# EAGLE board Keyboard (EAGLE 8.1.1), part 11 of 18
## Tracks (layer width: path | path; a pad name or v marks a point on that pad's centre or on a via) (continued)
S$11029 (continued)
  Bottom 0: 44.44,41.74 44.79,41.73
S$11030
  Bottom 0: 44.79,41.73 45.13,41.79
S$11031
  Bottom 0: 45.13,41.79 45.31,41.88
S$11032
  Bottom 0: 45.31,41.88 51,36.2
S$11033
  Bottom 0: 51,36.2 51.05,36.16
S$11034
  Bottom 0: 51.05,36.16 51.11,36.12
S$11035
  Bottom 0: 51.11,36.12 51.17,36.09
S$11036
  Bottom 0: 51.17,36.09 51.24,36.08
S$11037
  Bottom 0: 51.24,36.08 51.31,36.07
S$11038
  Bottom 0: 51.31,36.07 53.88,36.07
S$11039
  Bottom 0: 53.88,36.07 53.83,36.06
S$11040
  Bottom 0: 53.83,36.06 53.54,35.91
S$11041
  Bottom 0: 53.54,35.91 53.31,35.69
S$11042
  Bottom 0: 53.31,35.69 53.13,35.41
S$11043
  Bottom 0: 53.13,35.41 53.05,35.1
S$11044
  Bottom 0: 53.05,35.1 53.05,34.77
S$11045
  Bottom 0: 53.05,34.77 53.13,34.46
S$11046
  Bottom 0: 53.13,34.46 53.31,34.19
S$11047
  Bottom 0: 53.31,34.19 53.54,33.96
S$11048
  Bottom 0: 53.54,33.96 53.83,33.81
S$11049
  Bottom 0: 53.83,33.81 54.15,33.75
S$11050
  Bottom 0: 54.15,33.75 54.48,33.77
S$11051
  Bottom 0: 54.48,33.77 54.57,33.8
S$11052
  Bottom 0: 54.57,33.8 57.92,30.45
S$11053
  Bottom 0: 57.92,30.45 57.92,18.78
S$11054
  Bottom 0: 57.92,18.78 57.92,18.69
S$11055
  Bottom 0: 57.92,18.69 57.95,18.6
S$11056
  Bottom 0: 57.95,18.6 57.98,18.52
S$11057
  Bottom 0: 57.98,18.52 58.03,18.44
S$11058
  Bottom 0: 58.03,18.44 58.09,18.38
S$11059
  Bottom 0: 58.09,18.38 60.24,16.22
S$11060
  Bottom 0: 60.24,16.22 60.2,16.05
S$11061
  Bottom 0: 60.2,16.05 60.2,15.72
S$11062
  Bottom 0: 60.2,15.72 60.28,15.41
S$11063
  Bottom 0: 60.28,15.41 60.45,15.14
S$11064
  Bottom 0: 60.45,15.14 60.69,14.91
S$11065
  Bottom 0: 60.69,14.91 60.81,14.85
S$11066
  Bottom 0: 60.81,14.85 60.81,13.35
S$11067
  Bottom 0: 60.81,13.35 59.95,12.5
S$11068
  Bottom 0: 48.26,30.54 50.03,30.54
S$11069
  Bottom 0: 50.03,30.54 50.11,30.55
S$11070
  Bottom 0: 50.11,30.55 50.18,30.59
S$11071
  Bottom 0: 50.18,30.59 50.24,30.65
S$11072
  Bottom 0: 50.24,30.65 50.28,30.72
S$11073
  Bottom 0: 50.28,30.72 50.29,30.8
S$11074
  Bottom 0: 50.29,30.8 50.29,32.58
S$11075
  Bottom 0: 50.29,32.58 50.28,32.65
S$11076
  Bottom 0: 50.28,32.65 50.24,32.72
S$11077
  Bottom 0: 50.24,32.72 50.18,32.78
S$11078
  Bottom 0: 50.18,32.78 50.11,32.82
S$11079
  Bottom 0: 50.11,32.82 50.03,32.83
S$11080
  Bottom 0: 50.03,32.83 49.59,32.83
S$11081
  Bottom 0: 49.59,32.83 49.59,32.96
S$11082
  Bottom 0: 49.59,32.96 49.53,33.18
S$11083
  Bottom 0: 49.53,33.18 49.37,33.34
S$11084
  Bottom 0: 49.37,33.34 49.15,33.4
S$11085
  Bottom 0: 49.15,33.4 48.78,33.4
S$11086
  Bottom 0: 48.78,33.4 47.7,34.48
S$11087
  Bottom 0: 47.7,34.48 47.76,34.62
S$11088
  Bottom 0: 47.76,34.62 47.8,34.94
S$11089
  Bottom 0: 47.8,34.94 47.76,35.26
S$11090
  Bottom 0: 47.76,35.26 47.63,35.56
S$11091
  Bottom 0: 47.63,35.56 47.42,35.81
S$11092
  Bottom 0: 47.42,35.81 47.16,36
S$11093
  Bottom 0: 47.16,36 46.85,36.11
S$11094
  Bottom 0: 46.85,36.11 46.53,36.13
S$11095
  Bottom 0: 46.53,36.13 46.21,36.06
S$11096
  Bottom 0: 46.21,36.06 45.92,35.91
S$11097
  Bottom 0: 45.92,35.91 45.69,35.69
S$11098
  Bottom 0: 45.69,35.69 45.51,35.41
S$11099
  Bottom 0: 45.51,35.41 45.43,35.1
S$11100
  Bottom 0: 45.43,35.1 45.43,34.77
S$11101
  Bottom 0: 45.43,34.77 45.51,34.46
S$11102
  Bottom 0: 45.51,34.46 45.69,34.19
S$11103
  Bottom 0: 45.69,34.19 45.92,33.96
S$11104
  Bottom 0: 45.92,33.96 46.21,33.81
S$11105
  Bottom 0: 46.21,33.81 46.53,33.75
S$11106
  Bottom 0: 46.53,33.75 46.85,33.77
S$11107
  Bottom 0: 46.85,33.77 47.07,33.85
S$11108
  Bottom 0: 47.07,33.85 48.13,32.79
S$11109
  Bottom 0: 48.13,32.79 48.11,32.78
S$11110
  Bottom 0: 48.11,32.78 48.05,32.72
S$11111
  Bottom 0: 48.05,32.72 48.01,32.65
S$11112
  Bottom 0: 48.01,32.65 48,32.58
S$11113
  Bottom 0: 48,32.58 48,30.8
S$11114
  Bottom 0: 48,30.8 48.01,30.72
S$11115
  Bottom 0: 48.01,30.72 48.05,30.65
S$11116
  Bottom 0: 48.05,30.65 48.11,30.59
S$11117
  Bottom 0: 48.11,30.59 48.18,30.55
S$11118
  Bottom 0: 48.18,30.55 48.26,30.54
S$11119
  Bottom 0: 57.49,39.19 57.84,39.25
S$11120
  Bottom 0: 57.84,39.25 58.15,39.4
S$11121
  Bottom 0: 58.15,39.4 58.42,39.62
S$11122
  Bottom 0: 58.42,39.62 58.63,39.91
S$11123
  Bottom 0: 58.63,39.91 58.76,40.23
S$11124
  Bottom 0: 58.76,40.23 58.8,40.58
S$11125
  Bottom 0: 58.8,40.58 58.76,40.92
S$11126
  Bottom 0: 58.76,40.92 58.63,41.25
S$11127
  Bottom 0: 58.63,41.25 58.42,41.53
S$11128
  Bottom 0: 58.42,41.53 58.15,41.76
S$11129
  Bottom 0: 58.15,41.76 57.84,41.91
S$11130
  Bottom 0: 57.84,41.91 57.49,41.97
S$11131
  Bottom 0: 57.49,41.97 57.14,41.95
S$11132
  Bottom 0: 57.14,41.95 56.81,41.84
S$11133
  Bottom 0: 56.81,41.84 56.78,41.82
S$11134
  Bottom 0: 56.78,41.82 56.2,42.4
S$11135
  Bottom 0: 56.2,42.4 56.16,42.43
S$11136
  Bottom 0: 56.16,42.43 56.1,42.48
S$11137
  Bottom 0: 56.1,42.48 56.03,42.5
S$11138
  Bottom 0: 56.03,42.5 55.97,42.52
S$11139
  Bottom 0: 55.97,42.52 55.9,42.52
S$11140
  Bottom 0: 55.9,42.52 51.33,42.52
S$11141
  Bottom 0: 51.33,42.52 51.26,42.65
S$11142
  Bottom 0: 51.26,42.65 51.06,42.87
S$11143
  Bottom 0: 51.06,42.87 50.79,43.02
S$11144
  Bottom 0: 50.79,43.02 50.49,43.09
S$11145
  Bottom 0: 50.49,43.09 50.19,43.07
S$11146
  Bottom 0: 50.19,43.07 49.91,42.96
S$11147
  Bottom 0: 49.91,42.96 49.67,42.77
S$11148
  Bottom 0: 49.67,42.77 49.51,42.52
S$11149
  Bottom 0: 49.51,42.52 49.41,42.23
S$11150
  Bottom 0: 49.41,42.23 49.41,41.92
S$11151
  Bottom 0: 49.41,41.92 49.51,41.64
S$11152
  Bottom 0: 49.51,41.64 49.67,41.39
S$11153
  Bottom 0: 49.67,41.39 49.91,41.2
S$11154
  Bottom 0: 49.91,41.2 50.19,41.09
S$11155
  Bottom 0: 50.19,41.09 50.49,41.07
S$11156
  Bottom 0: 50.49,41.07 50.79,41.13
S$11157
  Bottom 0: 50.79,41.13 51.06,41.28
S$11158
  Bottom 0: 51.06,41.28 51.26,41.51
S$11159
  Bottom 0: 51.26,41.51 51.33,41.64
S$11160
  Bottom 0: 51.33,41.64 55.72,41.64
S$11161
  Bottom 0: 55.72,41.64 56.16,41.19
S$11162
  Bottom 0: 56.16,41.19 56.11,41.09
S$11163
  Bottom 0: 56.11,41.09 56.02,40.75
S$11164
  Bottom 0: 56.02,40.75 56.02,40.4
S$11165
  Bottom 0: 56.02,40.4 56.11,40.06
S$11166
  Bottom 0: 56.11,40.06 56.28,39.75
S$11167
  Bottom 0: 56.28,39.75 56.52,39.5
S$11168
  Bottom 0: 56.52,39.5 56.81,39.31
S$11169
  Bottom 0: 56.81,39.31 57.14,39.2
S$11170
  Bottom 0: 57.14,39.2 57.49,39.19
S$11171
  Bottom 0: 83.84,60.12 84.13,60.19
S$11172
  Bottom 0: 84.13,60.19 84.4,60.34
S$11173
  Bottom 0: 84.4,60.34 84.6,60.56
S$11174
  Bottom 0: 84.6,60.56 84.73,60.83
S$11175
  Bottom 0: 84.73,60.83 84.78,61.13
S$11176
  Bottom 0: 84.78,61.13 84.73,61.43
S$11177
  Bottom 0: 84.73,61.43 84.6,61.7
S$11178
  Bottom 0: 84.6,61.7 84.4,61.92
S$11179
  Bottom 0: 84.4,61.92 84.13,62.08
S$11180
  Bottom 0: 84.13,62.08 83.84,62.14
S$11181
  Bottom 0: 83.84,62.14 83.53,62.12
S$11182
  Bottom 0: 83.53,62.12 83.25,62.01
S$11183
  Bottom 0: 83.25,62.01 83.02,61.82
S$11184
  Bottom 0: 83.02,61.82 82.84,61.57
S$11185
  Bottom 0: 82.84,61.57 82.75,61.28
S$11186
  Bottom 0: 82.75,61.28 82.75,60.98
S$11187
  Bottom 0: 82.75,60.98 82.84,60.69
S$11188
  Bottom 0: 82.84,60.69 83.02,60.44
S$11189
  Bottom 0: 83.02,60.44 83.25,60.25
S$11190
  Bottom 0: 83.25,60.25 83.53,60.14
S$11191
  Bottom 0: 83.53,60.14 83.84,60.12
S$11192
  Bottom 0: 72.07,68.64 73.85,68.64
S$11193
  Bottom 0: 73.85,68.64 73.92,68.65
S$11194
  Bottom 0: 73.92,68.65 74,68.69
S$11195
  Bottom 0: 74,68.69 74.05,68.75
S$11196
  Bottom 0: 74.05,68.75 74.09,68.82
S$11197
  Bottom 0: 74.09,68.82 74.11,68.9
S$11198
  Bottom 0: 74.11,68.9 74.11,70.67
S$11199
  Bottom 0: 74.11,70.67 74.09,70.75
S$11200
  Bottom 0: 74.09,70.75 74.05,70.82
S$11201
  Bottom 0: 74.05,70.82 74,70.88
S$11202
  Bottom 0: 74,70.88 73.92,70.92
S$11203
  Bottom 0: 73.92,70.92 73.85,70.93
S$11204
  Bottom 0: 73.85,70.93 73.4,70.93
S$11205
  Bottom 0: 73.4,70.93 73.4,71.06
S$11206
  Bottom 0: 73.4,71.06 73.34,71.28
S$11207
  Bottom 0: 73.34,71.28 73.18,71.44
S$11208
  Bottom 0: 73.18,71.44 72.96,71.5
S$11209
  Bottom 0: 72.96,71.5 72.6,71.5
S$11210
  Bottom 0: 72.6,71.5 71.51,72.58
S$11211
  Bottom 0: 71.51,72.58 71.57,72.72
S$11212
  Bottom 0: 71.57,72.72 71.62,73.04
S$11213
  Bottom 0: 71.62,73.04 71.57,73.36
S$11214
  Bottom 0: 71.57,73.36 71.44,73.66
S$11215
  Bottom 0: 71.44,73.66 71.24,73.92
S$11216
  Bottom 0: 71.24,73.92 70.97,74.11
S$11217
  Bottom 0: 70.97,74.11 70.67,74.21
S$11218
  Bottom 0: 70.67,74.21 70.34,74.23
S$11219
  Bottom 0: 70.34,74.23 70.03,74.17
S$11220
  Bottom 0: 70.03,74.17 69.73,74.02
S$11221
  Bottom 0: 69.73,74.02 69.5,73.8
S$11222
  Bottom 0: 69.5,73.8 69.33,73.52
S$11223
  Bottom 0: 69.33,73.52 69.24,73.2
S$11224
  Bottom 0: 69.24,73.2 69.24,72.88
S$11225
  Bottom 0: 69.24,72.88 69.33,72.56
S$11226
  Bottom 0: 69.33,72.56 69.5,72.29
S$11227
  Bottom 0: 69.5,72.29 69.73,72.07
S$11228
  Bottom 0: 69.73,72.07 70.03,71.92
S$11229
  Bottom 0: 70.03,71.92 70.34,71.85
S$11230
  Bottom 0: 70.34,71.85 70.67,71.87
S$11231
  Bottom 0: 70.67,71.87 70.89,71.95
S$11232
  Bottom 0: 70.89,71.95 71.95,70.89
S$11233
  Bottom 0: 71.95,70.89 71.92,70.88
S$11234
  Bottom 0: 71.92,70.88 71.87,70.82
S$11235
  Bottom 0: 71.87,70.82 71.83,70.75
S$11236
  Bottom 0: 71.83,70.75 71.82,70.67
S$11237
  Bottom 0: 71.82,70.67 71.82,68.9
S$11238
  Bottom 0: 71.82,68.9 71.83,68.82
S$11239
  Bottom 0: 71.83,68.82 71.87,68.75
S$11240
  Bottom 0: 71.87,68.75 71.92,68.69
S$11241
  Bottom 0: 71.92,68.69 72,68.65
S$11242
  Bottom 0: 72,68.65 72.07,68.64
S$11243
  Bottom 0: 75.34,68.65 75.66,68.65
S$11244
  Bottom 0: 75.66,68.65 75.97,68.75
S$11245
  Bottom 0: 75.97,68.75 76.25,68.92
S$11246
  Bottom 0: 76.25,68.92 76.46,69.16
S$11247
  Bottom 0: 76.46,69.16 76.6,69.47
S$11248
  Bottom 0: 76.6,69.47 76.64,69.79
S$11249
  Bottom 0: 76.64,69.79 76.6,70.11
S$11250
  Bottom 0: 76.6,70.11 76.46,70.41
S$11251
  Bottom 0: 76.46,70.41 76.25,70.65
S$11252
  Bottom 0: 76.25,70.65 75.97,70.83
S$11253
  Bottom 0: 75.97,70.83 75.66,70.92
S$11254
  Bottom 0: 75.66,70.92 75.34,70.92
S$11255
  Bottom 0: 75.34,70.92 75.03,70.83
S$11256
  Bottom 0: 75.03,70.83 74.75,70.65
S$11257
  Bottom 0: 74.75,70.65 74.54,70.41
S$11258
  Bottom 0: 74.54,70.41 74.4,70.11
S$11259
  Bottom 0: 74.4,70.11 74.36,69.79
S$11260
  Bottom 0: 74.36,69.79 74.4,69.47
S$11261
  Bottom 0: 74.4,69.47 74.54,69.16
S$11262
  Bottom 0: 74.54,69.16 74.75,68.92
S$11263
  Bottom 0: 74.75,68.92 75.03,68.75
S$11264
  Bottom 0: 75.03,68.75 75.34,68.65
S$11265
  Bottom 0: 226.65,12.6 226.66,12.64
S$11266
  Bottom 0: 226.66,12.64 226.62,12.96
S$11267
  Bottom 0: 226.62,12.96 226.48,13.26
S$11268
  Bottom 0: 226.48,13.26 226.27,13.5
S$11269
  Bottom 0: 226.27,13.5 225.99,13.68
S$11270
  Bottom 0: 225.99,13.68 225.68,13.77
S$11271
  Bottom 0: 225.68,13.77 225.57,13.77
S$11272
  Bottom 0: 225.57,13.77 219.4,19.94
S$11273
  Bottom 0: 219.4,19.94 219.34,20
S$11274
  Bottom 0: 219.34,20 219.26,20.04
S$11275
  Bottom 0: 219.26,20.04 219.18,20.08
S$11276
  Bottom 0: 219.18,20.08 219.09,20.1
S$11277
  Bottom 0: 219.09,20.1 219,20.1
S$11278
  Bottom 0: 219,20.1 218.91,20.1
S$11279
  Bottom 0: 218.91,20.1 218.76,20.25
S$11280
  Bottom 0: 218.76,20.25 219.06,20.16
S$11281
  Bottom 0: 219.06,20.16 219.41,20.14
S$11282
  Bottom 0: 219.41,20.14 219.76,20.2
S$11283
  Bottom 0: 219.76,20.2 220.07,20.35
S$11284
  Bottom 0: 220.07,20.35 220.34,20.57
S$11285
  Bottom 0: 220.34,20.57 220.55,20.86
S$11286
  Bottom 0: 220.55,20.86 220.68,21.18
S$11287
  Bottom 0: 220.68,21.18 220.72,21.53
S$11288
  Bottom 0: 220.72,21.53 220.68,21.87
S$11289
  Bottom 0: 220.68,21.87 220.55,22.2
S$11290
  Bottom 0: 220.55,22.2 220.34,22.48
S$11291
  Bottom 0: 220.34,22.48 220.07,22.7
S$11292
  Bottom 0: 220.07,22.7 219.76,22.86
S$11293
  Bottom 0: 219.76,22.86 219.41,22.92
S$11294
  Bottom 0: 219.41,22.92 219.06,22.9
S$11295
  Bottom 0: 219.06,22.9 218.73,22.79
S$11296
  Bottom 0: 218.73,22.79 218.44,22.6
S$11297
  Bottom 0: 218.44,22.6 218.23,22.38
S$11298
  Bottom 0: 218.23,22.38 218.23,25.98
S$11299
  Bottom 0: 218.23,25.98 219.78,27.53
S$11300
  Bottom 0: 219.78,27.53 219.75,27.48
S$11301
  Bottom 0: 219.75,27.48 219.63,27.05
S$11302
  Bottom 0: 219.63,27.05 219.58,26.61
S$11303
  Bottom 0: 219.58,26.61 219.63,26.16
S$11304
  Bottom 0: 219.63,26.16 219.75,25.73
S$11305
  Bottom 0: 219.75,25.73 219.97,25.34
S$11306
  Bottom 0: 219.97,25.34 220.25,24.99
S$11307
  Bottom 0: 220.25,24.99 220.6,24.71
S$11308
  Bottom 0: 220.6,24.71 220.99,24.49
S$11309
  Bottom 0: 220.99,24.49 221.42,24.37
S$11310
  Bottom 0: 221.42,24.37 221.87,24.32
S$11311
  Bottom 0: 221.87,24.32 222.31,24.37
S$11312
  Bottom 0: 222.31,24.37 222.74,24.49
S$11313
  Bottom 0: 222.74,24.49 223.14,24.71
S$11314
  Bottom 0: 223.14,24.71 223.48,24.99
S$11315
  Bottom 0: 223.48,24.99 223.77,25.34
S$11316
  Bottom 0: 223.77,25.34 223.98,25.73
S$11317
  Bottom 0: 223.98,25.73 224.11,26.16
S$11318
  Bottom 0: 224.11,26.16 224.15,26.61
S$11319
  Bottom 0: 224.15,26.61 224.11,27.05
S$11320
  Bottom 0: 224.11,27.05 223.98,27.48
S$11321
  Bottom 0: 223.98,27.48 223.77,27.88
S$11322
  Bottom 0: 223.77,27.88 223.48,28.22
S$11323
  Bottom 0: 223.48,28.22 223.14,28.51
S$11324
  Bottom 0: 223.14,28.51 222.74,28.72
S$11325
  Bottom 0: 222.74,28.72 222.31,28.85
S$11326
  Bottom 0: 222.31,28.85 221.87,28.89
S$11327
  Bottom 0: 221.87,28.89 221.42,28.85
S$11328
  Bottom 0: 221.42,28.85 220.99,28.72
S$11329
  Bottom 0: 220.99,28.72 220.94,28.69
S$11330
  Bottom 0: 220.94,28.69 222.84,30.59
S$11331
  Bottom 0: 222.84,30.59 222.97,30.55
S$11332
  Bottom 0: 222.97,30.55 223.3,30.55
S$11333
  Bottom 0: 223.3,30.55 223.61,30.64
S$11334
  Bottom 0: 223.61,30.64 223.88,30.82
S$11335
  Bottom 0: 223.88,30.82 224.1,31.07
S$11336
  Bottom 0: 224.1,31.07 224.23,31.37
S$11337
  Bottom 0: 224.23,31.37 224.28,31.69
S$11338
  Bottom 0: 224.28,31.69 224.23,32.01
S$11339
  Bottom 0: 224.23,32.01 224.1,32.31
S$11340
  Bottom 0: 224.1,32.31 223.88,32.55
S$11341
  Bottom 0: 223.88,32.55 223.61,32.73
S$11342
  Bottom 0: 223.61,32.73 223.56,32.74
S$11343
  Bottom 0: 223.56,32.74 223.56,33.17
S$11344
  Bottom 0: 223.56,33.17 223.56,33.16
S$11345
  Bottom 0: 223.56,33.16 223.6,33.1
S$11346
  Bottom 0: 223.6,33.1 225.23,31.47
S$11347
  Bottom 0: 225.23,31.47 225.23,25.38
S$11348
  Bottom 0: 225.23,25.38 225.08,25.33
S$11349
  Bottom 0: 225.08,25.33 224.79,25.14
S$11350
  Bottom 0: 224.79,25.14 224.55,24.89
S$11351
  Bottom 0: 224.55,24.89 224.37,24.58
S$11352
  Bottom 0: 224.37,24.58 224.29,24.24
S$11353
  Bottom 0: 224.29,24.24 224.29,23.89
S$11354
  Bottom 0: 224.29,23.89 224.37,23.55
S$11355
  Bottom 0: 224.37,23.55 224.55,23.24
S$11356
  Bottom 0: 224.55,23.24 224.79,22.99
S$11357
  Bottom 0: 224.79,22.99 225.08,22.8
S$11358
  Bottom 0: 225.08,22.8 225.41,22.7
S$11359
  Bottom 0: 225.41,22.7 225.76,22.68
S$11360
  Bottom 0: 225.76,22.68 226.11,22.74
S$11361
  Bottom 0: 226.11,22.74 226.42,22.89
S$11362
  Bottom 0: 226.42,22.89 226.69,23.11
S$11363
  Bottom 0: 226.69,23.11 226.9,23.4
S$11364
  Bottom 0: 226.9,23.4 227.03,23.72
S$11365
  Bottom 0: 227.03,23.72 227.07,24.07
S$11366
  Bottom 0: 227.07,24.07 227.03,24.41
S$11367
  Bottom 0: 227.03,24.41 226.9,24.74
S$11368
  Bottom 0: 226.9,24.74 226.69,25.02
S$11369
  Bottom 0: 226.69,25.02 226.42,25.25
S$11370
  Bottom 0: 226.42,25.25 226.12,25.39
S$11371
  Bottom 0: 226.12,25.39 226.12,31.66
S$11372
  Bottom 0: 226.12,31.66 226.11,31.73
S$11373
  Bottom 0: 226.11,31.73 226.1,31.8
S$11374
  Bottom 0: 226.1,31.8 226.07,31.86
S$11375
  Bottom 0: 226.07,31.86 226.03,31.92
S$11376
  Bottom 0: 226.03,31.92 225.99,31.98
S$11377
  Bottom 0: 225.99,31.98 224.36,33.61
S$11378
  Bottom 0: 224.36,33.61 224.36,36.37
S$11379
  Bottom 0: 224.36,36.37 224.43,36.42
S$11380
  Bottom 0: 224.43,36.42 224.56,36.63
S$11381
  Bottom 0: 224.56,36.63 224.6,36.88
S$11382
  Bottom 0: 224.6,36.88 224.56,37.13
S$11383
  Bottom 0: 224.56,37.13 224.43,37.34
S$11384
  Bottom 0: 224.43,37.34 224.22,37.49
S$11385
  Bottom 0: 224.22,37.49 223.98,37.56
S$11386
  Bottom 0: 223.98,37.56 223.73,37.54
S$11387
  Bottom 0: 223.73,37.54 223.56,37.45
S$11388
  Bottom 0: 223.56,37.45 223.56,38.8
S$11389
  Bottom 0: 223.56,38.8 223.55,38.9
S$11390
  Bottom 0: 223.55,38.9 223.53,38.98
S$11391
  Bottom 0: 223.53,38.98 223.5,39.06
S$11392
  Bottom 0: 223.5,39.06 223.45,39.14
S$11393
  Bottom 0: 223.45,39.14 223.39,39.2
S$11394
  Bottom 0: 223.39,39.2 221.4,41.19
S$11395
  Bottom 0: 221.4,41.19 221.66,41.09
S$11396
  Bottom 0: 221.66,41.09 221.96,41.07
S$11397
  Bottom 0: 221.96,41.07 222.21,41.12
S$11398
  Bottom 0: 222.21,41.12 223.08,40.26
S$11399
  Bottom 0: 223.08,40.26 223.13,40.22
S$11400
  Bottom 0: 223.13,40.22 223.19,40.18
S$11401
  Bottom 0: 223.19,40.18 223.25,40.16
S$11402
  Bottom 0: 223.25,40.16 223.32,40.14
S$11403
  Bottom 0: 223.32,40.14 223.39,40.13
S$11404
  Bottom 0: 223.39,40.13 227.53,40.13
S$11405
  Bottom 0: 227.53,40.13 227.55,40.06
S$11406
  Bottom 0: 227.55,40.06 227.72,39.75
S$11407
  Bottom 0: 227.72,39.75 227.96,39.5
S$11408
  Bottom 0: 227.96,39.5 228.26,39.31
S$11409
  Bottom 0: 228.26,39.31 228.59,39.2
S$11410
  Bottom 0: 228.59,39.2 228.94,39.19
S$11411
  Bottom 0: 228.94,39.19 229.28,39.25
S$11412
  Bottom 0: 229.28,39.25 229.6,39.4
S$11413
  Bottom 0: 229.6,39.4 229.87,39.62
S$11414
  Bottom 0: 229.87,39.62 230.08,39.91
S$11415
  Bottom 0: 230.08,39.91 230.2,40.23
S$11416
  Bottom 0: 230.2,40.23 230.25,40.58
S$11417
  Bottom 0: 230.25,40.58 230.2,40.92
S$11418
  Bottom 0: 230.2,40.92 230.08,41.25
S$11419
  Bottom 0: 230.08,41.25 229.87,41.53
S$11420
  Bottom 0: 229.87,41.53 229.6,41.76
S$11421
  Bottom 0: 229.6,41.76 229.28,41.91
S$11422
  Bottom 0: 229.28,41.91 228.94,41.97
S$11423
  Bottom 0: 228.94,41.97 228.59,41.95
S$11424
  Bottom 0: 228.59,41.95 228.26,41.84
S$11425
  Bottom 0: 228.26,41.84 227.96,41.65
S$11426
  Bottom 0: 227.96,41.65 227.72,41.4
S$11427
  Bottom 0: 227.72,41.4 227.55,41.09
S$11428
  Bottom 0: 227.55,41.09 227.53,41.02
S$11429
  Bottom 0: 227.53,41.02 223.58,41.02
S$11430
  Bottom 0: 223.58,41.02 222.84,41.76
S$11431
  Bottom 0: 222.84,41.76 222.86,41.78
S$11432
  Bottom 0: 222.86,41.78 222.9,42.08
S$11433
  Bottom 0: 222.9,42.08 222.86,42.38
S$11434
  Bottom 0: 222.86,42.38 222.72,42.65
S$11435
  Bottom 0: 222.72,42.65 222.52,42.87
S$11436
  Bottom 0: 222.52,42.87 222.26,43.02
S$11437
  Bottom 0: 222.26,43.02 221.96,43.09
S$11438
  Bottom 0: 221.96,43.09 221.66,43.07
S$11439
  Bottom 0: 221.66,43.07 221.38,42.96
S$11440
  Bottom 0: 221.38,42.96 221.14,42.77
S$11441
  Bottom 0: 221.14,42.77 220.97,42.52
S$11442
  Bottom 0: 220.97,42.52 220.88,42.23
S$11443
  Bottom 0: 220.88,42.23 220.88,41.92
S$11444
  Bottom 0: 220.88,41.92 220.97,41.64
S$11445
  Bottom 0: 220.97,41.64 221,41.59
S$11446
  Bottom 0: 221,41.59 217.79,44.8
S$11447
  Bottom 0: 217.79,44.8 217.79,47.12
S$11448
  Bottom 0: 217.79,47.12 217.79,47.22
S$11449
  Bottom 0: 217.79,47.22 217.76,47.3
S$11450
  Bottom 0: 217.76,47.3 217.73,47.38
S$11451
  Bottom 0: 217.73,47.38 217.69,47.46
S$11452
  Bottom 0: 217.69,47.46 217.62,47.53
S$11453
  Bottom 0: 217.62,47.53 214.71,50.43
S$11454
  Bottom 0: 214.71,50.43 214.75,50.74
S$11455
  Bottom 0: 214.75,50.74 214.71,51.06
S$11456
  Bottom 0: 214.71,51.06 214.57,51.36
S$11457
  Bottom 0: 214.57,51.36 214.36,51.6
S$11458
  Bottom 0: 214.36,51.6 214.08,51.78
S$11459
  Bottom 0: 214.08,51.78 213.77,51.87
S$11460
  Bottom 0: 213.77,51.87 213.45,51.87
S$11461
  Bottom 0: 213.45,51.87 213.14,51.78
S$11462
  Bottom 0: 213.14,51.78 212.87,51.6
S$11463
  Bottom 0: 212.87,51.6 212.65,51.36
S$11464
  Bottom 0: 212.65,51.36 212.51,51.06
S$11465
  Bottom 0: 212.51,51.06 212.47,50.74
S$11466
  Bottom 0: 212.47,50.74 212.51,50.42
S$11467
  Bottom 0: 212.51,50.42 212.65,50.11
S$11468
  Bottom 0: 212.65,50.11 212.87,49.87
S$11469
  Bottom 0: 212.87,49.87 213.14,49.7
S$11470
  Bottom 0: 213.14,49.7 213.45,49.6
S$11471
  Bottom 0: 213.45,49.6 213.77,49.6
S$11472
  Bottom 0: 213.77,49.6 213.9,49.64
S$11473
  Bottom 0: 213.9,49.64 216.65,46.89
S$11474
  Bottom 0: 216.65,46.89 216.65,44.57
S$11475
  Bottom 0: 216.65,44.57 216.66,44.48
S$11476
  Bottom 0: 216.66,44.48 216.68,44.4
S$11477
  Bottom 0: 216.68,44.4 216.59,44.44
S$11478
  Bottom 0: 216.59,44.44 216.59,45.24
S$11479
  Bottom 0: 216.59,45.24 216.59,45.32
S$11480
  Bottom 0: 216.59,45.32 216.57,45.38
S$11481
  Bottom 0: 216.57,45.38 216.55,45.44
S$11482
  Bottom 0: 216.55,45.44 216.51,45.5
S$11483
  Bottom 0: 216.51,45.5 216.47,45.56
S$11484
  Bottom 0: 216.47,45.56 213.65,48.37
S$11485
  Bottom 0: 213.65,48.37 213.6,48.41
S$11486
  Bottom 0: 213.6,48.41 213.53,48.46
S$11487
  Bottom 0: 213.53,48.46 213.47,48.48
S$11488
  Bottom 0: 213.47,48.48 213.41,48.5
S$11489
  Bottom 0: 213.41,48.5 213.34,48.5
S$11490
  Bottom 0: 213.34,48.5 206.52,48.5
S$11491
  Bottom 0: 206.52,48.5 197.68,57.35
S$11492
  Bottom 0: 197.68,57.35 197.62,57.39
S$11493
  Bottom 0: 197.62,57.39 197.56,57.42
S$11494
  Bottom 0: 197.56,57.42 197.5,57.45
S$11495
  Bottom 0: 197.5,57.45 197.43,57.47
S$11496
  Bottom 0: 197.43,57.47 197.36,57.47
S$11497
  Bottom 0: 197.36,57.47 178.6,57.47
S$11498
  Bottom 0: 178.6,57.47 174.54,61.54
S$11499
  Bottom 0: 174.54,61.54 174.64,61.82
S$11500
  Bottom 0: 174.64,61.82 174.69,62.17
S$11501
  Bottom 0: 174.69,62.17 174.64,62.51
S$11502
  Bottom 0: 174.64,62.51 174.52,62.84
S$11503
  Bottom 0: 174.52,62.84 174.31,63.12
S$11504
  Bottom 0: 174.31,63.12 174.13,63.27
S$11505
  Bottom 0: 174.13,63.27 175.71,63.27
S$11506
  Bottom 0: 175.71,63.27 176.99,61.99
S$11507
  Bottom 0: 176.99,61.99 177.04,61.95
S$11508
  Bottom 0: 177.04,61.95 177.1,61.91
S$11509
  Bottom 0: 177.1,61.91 177.16,61.89
S$11510
  Bottom 0: 177.16,61.89 177.23,61.87
S$11511
  Bottom 0: 177.23,61.87 177.3,61.86
S$11512
  Bottom 0: 177.3,61.86 178.33,61.86
S$11513
  Bottom 0: 178.33,61.86 178.27,61.82
S$11514
  Bottom 0: 178.27,61.82 178.11,61.57
S$11515
  Bottom 0: 178.11,61.57 178.01,61.28
S$11516
  Bottom 0: 178.01,61.28 178.01,60.98
S$11517
  Bottom 0: 178.01,60.98 178.11,60.69
S$11518
  Bottom 0: 178.11,60.69 178.27,60.44
S$11519
  Bottom 0: 178.27,60.44 178.51,60.25
S$11520
  Bottom 0: 178.51,60.25 178.79,60.14
S$11521
  Bottom 0: 178.79,60.14 179.09,60.12
S$11522
  Bottom 0: 179.09,60.12 179.39,60.19
S$11523
  Bottom 0: 179.39,60.19 179.66,60.34
S$11524
  Bottom 0: 179.66,60.34 179.86,60.56
S$11525
  Bottom 0: 179.86,60.56 179.92,60.69
S$11526
  Bottom 0: 179.92,60.69 184.3,60.69
S$11527
  Bottom 0: 184.3,60.69 184.74,60.24
S$11528
  Bottom 0: 184.74,60.24 184.69,60.14
S$11529
  Bottom 0: 184.69,60.14 184.6,59.8
S$11530
  Bottom 0: 184.6,59.8 184.6,59.45
S$11531
  Bottom 0: 184.6,59.45 184.69,59.11
S$11532
  Bottom 0: 184.69,59.11 184.86,58.8
S$11533
  Bottom 0: 184.86,58.8 185.1,58.55
S$11534
  Bottom 0: 185.1,58.55 185.4,58.36
S$11535
  Bottom 0: 185.4,58.36 185.73,58.26
S$11536
  Bottom 0: 185.73,58.26 186.07,58.23
S$11537
  Bottom 0: 186.07,58.23 186.42,58.3
S$11538
  Bottom 0: 186.42,58.3 186.74,58.45
S$11539
  Bottom 0: 186.74,58.45 187.01,58.67
S$11540
  Bottom 0: 187.01,58.67 187.22,58.96
S$11541
  Bottom 0: 187.22,58.96 187.34,59.28
S$11542
  Bottom 0: 187.34,59.28 187.39,59.63
S$11543
  Bottom 0: 187.39,59.63 187.34,59.97
S$11544
  Bottom 0: 187.34,59.97 187.22,60.3
S$11545
  Bottom 0: 187.22,60.3 187.01,60.58
S$11546
  Bottom 0: 187.01,60.58 186.74,60.8
S$11547
  Bottom 0: 186.74,60.8 186.42,60.96
S$11548
  Bottom 0: 186.42,60.96 186.07,61.02
S$11549
  Bottom 0: 186.07,61.02 185.73,61
S$11550
  Bottom 0: 185.73,61 185.4,60.89
S$11551
  Bottom 0: 185.4,60.89 185.37,60.87
S$11552
  Bottom 0: 185.37,60.87 184.8,61.45
S$11553
  Bottom 0: 184.8,61.45 184.74,61.48
S$11554
  Bottom 0: 184.74,61.48 184.68,61.53
S$11555
  Bottom 0: 184.68,61.53 184.62,61.55
S$11556
  Bottom 0: 184.62,61.55 184.56,61.57
S$11557
  Bottom 0: 184.56,61.57 184.49,61.57
S$11558
  Bottom 0: 184.49,61.57 179.92,61.57
S$11559
  Bottom 0: 179.92,61.57 179.86,61.7
S$11560
  Bottom 0: 179.86,61.7 179.71,61.86
S$11561
  Bottom 0: 179.71,61.86 190.99,61.86
S$11562
  Bottom 0: 190.99,61.86 191.04,61.65
S$11563
  Bottom 0: 191.04,61.65 191.21,61.34
S$11564
  Bottom 0: 191.21,61.34 191.45,61.09
S$11565
  Bottom 0: 191.45,61.09 191.75,60.9
S$11566
  Bottom 0: 191.75,60.9 192.08,60.8
S$11567
  Bottom 0: 192.08,60.8 192.43,60.77
S$11568
  Bottom 0: 192.43,60.77 192.77,60.84
S$11569
  Bottom 0: 192.77,60.84 193.09,60.99
S$11570
  Bottom 0: 193.09,60.99 193.36,61.21
S$11571
  Bottom 0: 193.36,61.21 193.57,61.5
S$11572
  Bottom 0: 193.57,61.5 193.69,61.82
S$11573
  Bottom 0: 193.69,61.82 193.74,62.17
S$11574
  Bottom 0: 193.74,62.17 193.69,62.51
S$11575
  Bottom 0: 193.69,62.51 193.57,62.84
S$11576
  Bottom 0: 193.57,62.84 193.36,63.12
S$11577
  Bottom 0: 193.36,63.12 193.09,63.34
S$11578
  Bottom 0: 193.09,63.34 192.78,63.49
S$11579
  Bottom 0: 192.78,63.49 192.78,64.65
S$11580
  Bottom 0: 192.78,64.65 197.08,68.95
S$11581
  Bottom 0: 197.08,68.95 197.06,68.9
S$11582
  Bottom 0: 197.06,68.9 197.06,68.59
S$11583
  Bottom 0: 197.06,68.59 197.16,68.31
S$11584
  Bottom 0: 197.16,68.31 197.32,68.06
S$11585
  Bottom 0: 197.32,68.06 197.56,67.87
S$11586
  Bottom 0: 197.56,67.87 197.84,67.76
S$11587
  Bottom 0: 197.84,67.76 198.15,67.74
S$11588
  Bottom 0: 198.15,67.74 198.39,67.8
S$11589
  Bottom 0: 198.39,67.8 205.18,61.01
S$11590
  Bottom 0: 205.18,61.01 205.12,61.02
S$11591
  Bottom 0: 205.12,61.02 204.78,61
S$11592
  Bottom 0: 204.78,61 204.45,60.89
S$11593
  Bottom 0: 204.45,60.89 204.42,60.87
S$11594
  Bottom 0: 204.42,60.87 203.84,61.45
S$11595
  Bottom 0: 203.84,61.45 203.79,61.48
S$11596
  Bottom 0: 203.79,61.48 203.73,61.53
S$11597
  Bottom 0: 203.73,61.53 203.67,61.55
S$11598
  Bottom 0: 203.67,61.55 203.6,61.57
S$11599
  Bottom 0: 203.6,61.57 203.53,61.57
S$11600
  Bottom 0: 203.53,61.57 198.97,61.57
S$11601
  Bottom 0: 198.97,61.57 198.91,61.7
S$11602
  Bottom 0: 198.91,61.7 198.71,61.92
S$11603
  Bottom 0: 198.71,61.92 198.44,62.08
S$11604
  Bottom 0: 198.44,62.08 198.15,62.14
S$11605
  Bottom 0: 198.15,62.14 197.84,62.12
S$11606
  Bottom 0: 197.84,62.12 197.56,62.01
S$11607
  Bottom 0: 197.56,62.01 197.32,61.82
S$11608
  Bottom 0: 197.32,61.82 197.16,61.57
S$11609
  Bottom 0: 197.16,61.57 197.06,61.28
S$11610
  Bottom 0: 197.06,61.28 197.06,60.98
S$11611
  Bottom 0: 197.06,60.98 197.16,60.69
S$11612
  Bottom 0: 197.16,60.69 197.32,60.44
S$11613
  Bottom 0: 197.32,60.44 197.56,60.25
S$11614
  Bottom 0: 197.56,60.25 197.84,60.14
S$11615
  Bottom 0: 197.84,60.14 198.15,60.12
S$11616
  Bottom 0: 198.15,60.12 198.44,60.19
S$11617
  Bottom 0: 198.44,60.19 198.71,60.34
S$11618
  Bottom 0: 198.71,60.34 198.91,60.56
S$11619
  Bottom 0: 198.91,60.56 198.97,60.69
S$11620
  Bottom 0: 198.97,60.69 203.35,60.69
S$11621
  Bottom 0: 203.35,60.69 203.79,60.24
S$11622
  Bottom 0: 203.79,60.24 203.74,60.14
S$11623
  Bottom 0: 203.74,60.14 203.66,59.8
S$11624
  Bottom 0: 203.66,59.8 203.66,59.45
S$11625
  Bottom 0: 203.66,59.45 203.74,59.11
S$11626
  Bottom 0: 203.74,59.11 203.91,58.8
S$11627
  Bottom 0: 203.91,58.8 204.15,58.55
S$11628
  Bottom 0: 204.15,58.55 204.45,58.36
S$11629
  Bottom 0: 204.45,58.36 204.78,58.26
S$11630
  Bottom 0: 204.78,58.26 205.12,58.23
S$11631
  Bottom 0: 205.12,58.23 205.47,58.3
S$11632
  Bottom 0: 205.47,58.3 205.79,58.45
S$11633
  Bottom 0: 205.79,58.45 206.06,58.67
S$11634
  Bottom 0: 206.06,58.67 206.27,58.96
S$11635
  Bottom 0: 206.27,58.96 206.39,59.28
S$11636
  Bottom 0: 206.39,59.28 206.44,59.63
S$11637
  Bottom 0: 206.44,59.63 206.42,59.77
S$11638
  Bottom 0: 206.42,59.77 223.95,42.24
S$11639
  Bottom 0: 223.95,42.24 224,42.2
S$11640
  Bottom 0: 224,42.2 224.07,42.16
S$11641
  Bottom 0: 224.07,42.16 224.13,42.14
S$11642
  Bottom 0: 224.13,42.14 224.19,42.12
S$11643
  Bottom 0: 224.19,42.12 224.26,42.11
S$11644
  Bottom 0: 224.26,42.11 232.72,42.11
S$11645
  Bottom 0: 232.72,42.11 233.54,41.29
S$11646
  Bottom 0: 233.54,41.29 233.6,41.25
S$11647
  Bottom 0: 233.6,41.25 233.66,41.21
S$11648
  Bottom 0: 233.66,41.21 233.72,41.19
S$11649
  Bottom 0: 233.72,41.19 233.78,41.17
S$11650
  Bottom 0: 233.78,41.17 233.85,41.16
S$11651
  Bottom 0: 233.85,41.16 235.85,41.16
S$11652
  Bottom 0: 235.85,41.16 235.92,41.17
S$11653
  Bottom 0: 235.92,41.17 235.98,41.19
S$11654
  Bottom 0: 235.98,41.19 236.04,41.21
S$11655
  Bottom 0: 236.04,41.21 236.11,41.25
S$11656
  Bottom 0: 236.11,41.25 236.16,41.29
S$11657
  Bottom 0: 236.16,41.29 242.93,48.06
S$11658
  Bottom 0: 242.93,48.06 242.97,48.12
S$11659
  Bottom 0: 242.97,48.12 243.01,48.17
S$11660
  Bottom 0: 243.01,48.17 243.04,48.24
S$11661
  Bottom 0: 243.04,48.24 243.06,48.3
S$11662
  Bottom 0: 243.06,48.3 243.06,48.35
S$11663
  Bottom 0: 243.06,48.35 243.13,48.4
S$11664
  Bottom 0: 243.13,48.4 243.26,48.62
S$11665
  Bottom 0: 243.26,48.62 243.3,48.87
S$11666
  Bottom 0: 243.3,48.87 243.26,49.12
S$11667
  Bottom 0: 243.26,49.12 243.25,49.13
S$11668
  Bottom 0: 243.25,49.13 243.47,49.18
S$11669
  Bottom 0: 243.47,49.18 243.52,49.22
S$11670
  Bottom 0: 243.52,49.22 243.52,29.46
S$11671
  Bottom 0: 243.52,29.46 226.65,12.6
S$11672
  Bottom 0: 228,14.7 228.33,14.72
S$11673
  Bottom 0: 228.33,14.72 228.63,14.83
S$11674
  Bottom 0: 228.63,14.83 228.9,15.01
S$11675
  Bottom 0: 228.9,15.01 229.1,15.27
S$11676
  Bottom 0: 229.1,15.27 229.23,15.57
S$11677
  Bottom 0: 229.23,15.57 229.28,15.89
S$11678
  Bottom 0: 229.28,15.89 229.23,16.21
S$11679
  Bottom 0: 229.23,16.21 229.1,16.51
S$11680
  Bottom 0: 229.1,16.51 228.9,16.76
S$11681
  Bottom 0: 228.9,16.76 228.65,16.93
S$11682
  Bottom 0: 228.65,16.93 228.65,28.03
S$11683
  Bottom 0: 228.65,28.03 229.89,29.27
S$11684
  Bottom 0: 229.89,29.27 230.14,29.22
S$11685
  Bottom 0: 230.14,29.22 230.46,29.24
S$11686
  Bottom 0: 230.46,29.24 230.77,29.35
S$11687
  Bottom 0: 230.77,29.35 231.03,29.54
S$11688
  Bottom 0: 231.03,29.54 231.24,29.79
S$11689
  Bottom 0: 231.24,29.79 231.37,30.09
S$11690
  Bottom 0: 231.37,30.09 231.41,30.41
S$11691
  Bottom 0: 231.41,30.41 231.37,30.73
S$11692
  Bottom 0: 231.37,30.73 231.24,31.03
S$11693
  Bottom 0: 231.24,31.03 231.03,31.29
S$11694
  Bottom 0: 231.03,31.29 230.77,31.47
S$11695
  Bottom 0: 230.77,31.47 230.46,31.58
S$11696
  Bottom 0: 230.46,31.58 230.14,31.6
S$11697
  Bottom 0: 230.14,31.6 229.89,31.55
S$11698
  Bottom 0: 229.89,31.55 226.84,34.6
S$11699
  Bottom 0: 226.84,34.6 226.85,34.62
S$11700
  Bottom 0: 226.85,34.62 226.9,34.94
S$11701
  Bottom 0: 226.9,34.94 226.85,35.26
S$11702
  Bottom 0: 226.85,35.26 226.72,35.56
S$11703
  Bottom 0: 226.72,35.56 226.51,35.81
S$11704
  Bottom 0: 226.51,35.81 226.25,36
S$11705
  Bottom 0: 226.25,36 225.95,36.11
S$11706
  Bottom 0: 225.95,36.11 225.62,36.13
S$11707
  Bottom 0: 225.62,36.13 225.3,36.06
S$11708
  Bottom 0: 225.3,36.06 225.01,35.91
S$11709
  Bottom 0: 225.01,35.91 224.78,35.69
S$11710
  Bottom 0: 224.78,35.69 224.6,35.41
S$11711
  Bottom 0: 224.6,35.41 224.52,35.1
S$11712
  Bottom 0: 224.52,35.1 224.52,34.77
S$11713
  Bottom 0: 224.52,34.77 224.6,34.46
S$11714
  Bottom 0: 224.6,34.46 224.78,34.19
S$11715
  Bottom 0: 224.78,34.19 225.01,33.96
S$11716
  Bottom 0: 225.01,33.96 225.3,33.81
S$11717
  Bottom 0: 225.3,33.81 225.62,33.75
S$11718
  Bottom 0: 225.62,33.75 225.95,33.77
S$11719
  Bottom 0: 225.95,33.77 226.04,33.8
S$11720
  Bottom 0: 226.04,33.8 229.09,30.75
S$11721
  Bottom 0: 229.09,30.75 229.04,30.57
S$11722
  Bottom 0: 229.04,30.57 229.04,30.25
S$11723
  Bottom 0: 229.04,30.25 229.09,30.08
S$11724
  Bottom 0: 229.09,30.08 227.68,28.67
S$11725
  Bottom 0: 227.68,28.67 227.62,28.6
S$11726
  Bottom 0: 227.62,28.6 227.58,28.53
S$11727
  Bottom 0: 227.58,28.53 227.54,28.45
S$11728
  Bottom 0: 227.54,28.45 227.52,28.35
S$11729
  Bottom 0: 227.52,28.35 227.51,28.27
S$11730
  Bottom 0: 227.51,28.27 227.51,16.92
S$11731
  Bottom 0: 227.51,16.92 227.39,16.86
S$11732
  Bottom 0: 227.39,16.86 227.16,16.64
S$11733
  Bottom 0: 227.16,16.64 226.99,16.36
S$11734
  Bottom 0: 226.99,16.36 226.9,16.05
S$11735
  Bottom 0: 226.9,16.05 226.9,15.72
S$11736
  Bottom 0: 226.9,15.72 226.99,15.41
S$11737
  Bottom 0: 226.99,15.41 227.16,15.14
S$11738
  Bottom 0: 227.16,15.14 227.39,14.91
S$11739
  Bottom 0: 227.39,14.91 227.68,14.77
S$11740
  Bottom 0: 227.68,14.77 228,14.7
S$11741
  Bottom 0: 230.14,21.6 230.46,21.62
S$11742
  Bottom 0: 230.46,21.62 230.77,21.73
S$11743
  Bottom 0: 230.77,21.73 231.03,21.92
S$11744
  Bottom 0: 231.03,21.92 231.24,22.17
S$11745
  Bottom 0: 231.24,22.17 231.32,22.35
S$11746
  Bottom 0: 231.32,22.35 233.03,22.35
S$11747
  Bottom 0: 233.03,22.35 233.1,22.36
S$11748
  Bottom 0: 233.1,22.36 233.17,22.37
S$11749
  Bottom 0: 233.17,22.37 233.23,22.39
S$11750
  Bottom 0: 233.23,22.39 233.29,22.44
S$11751
  Bottom 0: 233.29,22.44 233.35,22.48
S$11752
  Bottom 0: 233.35,22.48 241.89,31.02
S$11753
  Bottom 0: 241.89,31.02 241.99,31.01
S$11754
  Bottom 0: 241.99,31.01 242.23,31.07
S$11755
  Bottom 0: 242.23,31.07 242.44,31.22
S$11756
  Bottom 0: 242.44,31.22 242.57,31.44
S$11757
  Bottom 0: 242.57,31.44 242.61,31.69
S$11758
  Bottom 0: 242.61,31.69 242.57,31.93
S$11759
  Bottom 0: 242.57,31.93 242.44,32.15
S$11760
  Bottom 0: 242.44,32.15 242.23,32.3
S$11761
  Bottom 0: 242.23,32.3 241.99,32.37
S$11762
  Bottom 0: 241.99,32.37 241.74,32.35
S$11763
  Bottom 0: 241.74,32.35 241.51,32.23
S$11764
  Bottom 0: 241.51,32.23 241.34,32.05
S$11765
  Bottom 0: 241.34,32.05 241.25,31.81
S$11766
  Bottom 0: 241.25,31.81 241.25,31.64
S$11767
  Bottom 0: 241.25,31.64 232.84,23.23
S$11768
  Bottom 0: 232.84,23.23 231.32,23.23
S$11769
  Bottom 0: 231.32,23.23 231.24,23.41
S$11770
  Bottom 0: 231.24,23.41 231.03,23.66
S$11771
  Bottom 0: 231.03,23.66 230.77,23.85
S$11772
  Bottom 0: 230.77,23.85 230.46,23.96
S$11773
  Bottom 0: 230.46,23.96 230.14,23.98
S$11774
  Bottom 0: 230.14,23.98 229.82,23.91
S$11775
  Bottom 0: 229.82,23.91 229.53,23.77
S$11776
  Bottom 0: 229.53,23.77 229.3,23.54
S$11777
  Bottom 0: 229.3,23.54 229.13,23.27
S$11778
  Bottom 0: 229.13,23.27 229.04,22.95
S$11779
  Bottom 0: 229.04,22.95 229.04,22.63
S$11780
  Bottom 0: 229.04,22.63 229.13,22.31
S$11781
  Bottom 0: 229.13,22.31 229.3,22.04
S$11782
  Bottom 0: 229.3,22.04 229.53,21.82
S$11783
  Bottom 0: 229.53,21.82 229.82,21.67
S$11784
  Bottom 0: 229.82,21.67 230.14,21.6
S$11785
  Bottom 0: 241.02,41.07 241.31,41.13
S$11786
  Bottom 0: 241.31,41.13 241.57,41.28
S$11787
  Bottom 0: 241.57,41.28 241.78,41.51
S$11788
  Bottom 0: 241.78,41.51 241.91,41.78
S$11789
  Bottom 0: 241.91,41.78 241.96,42.08
S$11790
  Bottom 0: 241.96,42.08 241.91,42.38
S$11791
  Bottom 0: 241.91,42.38 241.78,42.65
S$11792
  Bottom 0: 241.78,42.65 241.57,42.87
S$11793
  Bottom 0: 241.57,42.87 241.31,43.02
S$11794
  Bottom 0: 241.31,43.02 241.02,43.09
S$11795
  Bottom 0: 241.02,43.09 240.71,43.07
S$11796
  Bottom 0: 240.71,43.07 240.43,42.96
S$11797
  Bottom 0: 240.43,42.96 240.19,42.77
S$11798
  Bottom 0: 240.19,42.77 240.03,42.52
S$11799
  Bottom 0: 240.03,42.52 239.94,42.23
S$11800
  Bottom 0: 239.94,42.23 239.94,41.92
S$11801
  Bottom 0: 239.94,41.92 240.03,41.64
S$11802
  Bottom 0: 240.03,41.64 240.19,41.39
S$11803
  Bottom 0: 240.19,41.39 240.43,41.2
S$11804
  Bottom 0: 240.43,41.2 240.71,41.09
S$11805
  Bottom 0: 240.71,41.09 241.02,41.07
S$11806
  Bottom 0: 210.18,49.59 211.96,49.59
S$11807
  Bottom 0: 211.96,49.59 212.04,49.6
S$11808
  Bottom 0: 212.04,49.6 212.11,49.64
S$11809
  Bottom 0: 212.11,49.64 212.16,49.7
S$11810
  Bottom 0: 212.16,49.7 212.2,49.77
S$11811
  Bottom 0: 212.2,49.77 212.21,49.85
S$11812
  Bottom 0: 212.21,49.85 212.21,51.63
S$11813
  Bottom 0: 212.21,51.63 212.2,51.7
S$11814
  Bottom 0: 212.2,51.7 212.16,51.77
S$11815
  Bottom 0: 212.16,51.77 212.11,51.83
S$11816
  Bottom 0: 212.11,51.83 212.04,51.87
S$11817
  Bottom 0: 212.04,51.87 211.96,51.88
S$11818
  Bottom 0: 211.96,51.88 211.51,51.88
S$11819
  Bottom 0: 211.51,51.88 211.51,52.01
S$11820
  Bottom 0: 211.51,52.01 211.45,52.23
S$11821
  Bottom 0: 211.45,52.23 211.29,52.39
S$11822
  Bottom 0: 211.29,52.39 211.07,52.45
S$11823
  Bottom 0: 211.07,52.45 210.72,52.45
S$11824
  Bottom 0: 210.72,52.45 209.64,53.52
S$11825
  Bottom 0: 209.64,53.52 209.7,53.67
S$11826
  Bottom 0: 209.7,53.67 209.75,53.98
S$11827
  Bottom 0: 209.75,53.98 209.7,54.3
S$11828
  Bottom 0: 209.7,54.3 209.57,54.61
S$11829
  Bottom 0: 209.57,54.61 209.37,54.86
S$11830
  Bottom 0: 209.37,54.86 209.1,55.05
S$11831
  Bottom 0: 209.1,55.05 208.8,55.16
S$11832
  Bottom 0: 208.8,55.16 208.47,55.18
S$11833
  Bottom 0: 208.47,55.18 208.15,55.11
S$11834
  Bottom 0: 208.15,55.11 207.86,54.96
S$11835
  Bottom 0: 207.86,54.96 207.63,54.74
S$11836
  Bottom 0: 207.63,54.74 207.45,54.47
S$11837
  Bottom 0: 207.45,54.47 207.37,54.15
S$11838
  Bottom 0: 207.37,54.15 207.37,53.83
S$11839
  Bottom 0: 207.37,53.83 207.45,53.51
S$11840
  Bottom 0: 207.45,53.51 207.63,53.23
S$11841
  Bottom 0: 207.63,53.23 207.86,53.01
S$11842
  Bottom 0: 207.86,53.01 208.15,52.87
S$11843
  Bottom 0: 208.15,52.87 208.47,52.8
S$11844
  Bottom 0: 208.47,52.8 208.8,52.82
S$11845
  Bottom 0: 208.8,52.82 209.02,52.9
S$11846
  Bottom 0: 209.02,52.9 210.07,51.85
S$11847
  Bottom 0: 210.07,51.85 210.03,51.83
S$11848
  Bottom 0: 210.03,51.83 209.98,51.77
S$11849
  Bottom 0: 209.98,51.77 209.94,51.7
S$11850
  Bottom 0: 209.94,51.7 209.93,51.63
S$11851
  Bottom 0: 209.93,51.63 209.93,49.85
S$11852
  Bottom 0: 209.93,49.85 209.94,49.77
S$11853
  Bottom 0: 209.94,49.77 209.98,49.7
S$11854
  Bottom 0: 209.98,49.7 210.03,49.64
S$11855
  Bottom 0: 210.03,49.64 210.11,49.6
S$11856
  Bottom 0: 210.11,49.6 210.18,49.59
S$11857
  Bottom 0: 12.19,13.21 12.17,13.26
S$11858
  Bottom 0: 12.17,13.26 11.95,13.5
S$11859
  Bottom 0: 11.95,13.5 11.68,13.68
S$11860
  Bottom 0: 11.68,13.68 11.37,13.77
S$11861
  Bottom 0: 11.37,13.77 11.05,13.77
S$11862
  Bottom 0: 11.05,13.77 10.73,13.68
S$11863
  Bottom 0: 10.73,13.68 10.46,13.5
S$11864
  Bottom 0: 10.46,13.5 10.37,13.39
S$11865
  Bottom 0: 10.37,13.39 10.37,34.35
S$11866
  Bottom 0: 10.37,34.35 17.89,41.86
S$11867
  Bottom 0: 17.89,41.86 17.91,41.85
S$11868
  Bottom 0: 17.91,41.85 18.24,41.74
S$11869
  Bottom 0: 18.24,41.74 18.59,41.73
S$11870
  Bottom 0: 18.59,41.73 18.94,41.79
S$11871
  Bottom 0: 18.94,41.79 19.26,41.94
S$11872
  Bottom 0: 19.26,41.94 19.52,42.16
S$11873
  Bottom 0: 19.52,42.16 19.68,42.38
S$11874
  Bottom 0: 19.68,42.38 19.68,40.49
S$11875
  Bottom 0: 19.68,40.49 17.65,38.45
S$11876
  Bottom 0: 17.65,38.45 17.56,38.48
S$11877
  Bottom 0: 17.56,38.48 17.24,38.5
S$11878
  Bottom 0: 17.24,38.5 16.92,38.44
S$11879
  Bottom 0: 16.92,38.44 16.63,38.29
S$11880
  Bottom 0: 16.63,38.29 16.4,38.07
S$11881
  Bottom 0: 16.4,38.07 16.22,37.79
S$11882
  Bottom 0: 16.22,37.79 16.13,37.48
S$11883
  Bottom 0: 16.13,37.48 16.13,37.15
S$11884
  Bottom 0: 16.13,37.15 16.22,36.84
S$11885
  Bottom 0: 16.22,36.84 16.4,36.56
S$11886
  Bottom 0: 16.4,36.56 16.63,36.34
S$11887
  Bottom 0: 16.63,36.34 16.92,36.19
S$11888
  Bottom 0: 16.92,36.19 17.24,36.13
S$11889
  Bottom 0: 17.24,36.13 17.56,36.15
S$11890
  Bottom 0: 17.56,36.15 17.87,36.25
S$11891
  Bottom 0: 17.87,36.25 18.13,36.44
S$11892
  Bottom 0: 18.13,36.44 18.34,36.7
S$11893
  Bottom 0: 18.34,36.7 18.47,36.99
S$11894
  Bottom 0: 18.47,36.99 18.51,37.31
S$11895
  Bottom 0: 18.51,37.31 18.47,37.63
S$11896
  Bottom 0: 18.47,37.63 18.46,37.66
S$11897
  Bottom 0: 18.46,37.66 20.66,39.85
S$11898
  Bottom 0: 20.66,39.85 20.72,39.92
S$11899
  Bottom 0: 20.72,39.92 20.77,40
S$11900
  Bottom 0: 20.77,40 20.8,40.08
S$11901
  Bottom 0: 20.8,40.08 20.82,40.16
S$11902
  Bottom 0: 20.82,40.16 20.82,40.26
S$11903
  Bottom 0: 20.82,40.26 20.82,45.55
S$11904
  Bottom 0: 20.82,45.55 20.82,45.65
S$11905
  Bottom 0: 20.82,45.65 20.8,45.73
S$11906
  Bottom 0: 20.8,45.73 20.77,45.81
S$11907
  Bottom 0: 20.77,45.81 20.72,45.89
S$11908
  Bottom 0: 20.72,45.89 20.66,45.96
S$11909
  Bottom 0: 20.66,45.96 17.38,49.24
S$11910
  Bottom 0: 17.38,49.24 17.9,49.77
S$11911
  Bottom 0: 17.9,49.77 17.96,49.83
S$11912
  Bottom 0: 17.96,49.83 18.01,49.91
S$11913
  Bottom 0: 18.01,49.91 18.04,49.99
S$11914
  Bottom 0: 18.04,49.99 18.07,50.08
S$11915
  Bottom 0: 18.07,50.08 18.07,50.17
S$11916
  Bottom 0: 18.07,50.17 18.07,53.07
S$11917
  Bottom 0: 18.07,53.07 18.13,53.11
S$11918
  Bottom 0: 18.13,53.11 18.34,53.37
S$11919
  Bottom 0: 18.34,53.37 18.47,53.67
S$11920
  Bottom 0: 18.47,53.67 18.51,53.98
S$11921
  Bottom 0: 18.51,53.98 18.47,54.3
S$11922
  Bottom 0: 18.47,54.3 18.34,54.61
S$11923
  Bottom 0: 18.34,54.61 18.13,54.86
S$11924
  Bottom 0: 18.13,54.86 17.87,55.05
S$11925
  Bottom 0: 17.87,55.05 17.56,55.16
S$11926
  Bottom 0: 17.56,55.16 17.24,55.18
S$11927
  Bottom 0: 17.24,55.18 16.92,55.11
S$11928
  Bottom 0: 16.92,55.11 16.63,54.96
S$11929
  Bottom 0: 16.63,54.96 16.4,54.74
S$11930
  Bottom 0: 16.4,54.74 16.22,54.47
S$11931
  Bottom 0: 16.22,54.47 16.13,54.15
S$11932
  Bottom 0: 16.13,54.15 16.13,53.83
S$11933
  Bottom 0: 16.13,53.83 16.22,53.51
S$11934
  Bottom 0: 16.22,53.51 16.4,53.23
S$11935
  Bottom 0: 16.4,53.23 16.63,53.01
S$11936
  Bottom 0: 16.63,53.01 16.92,52.87
S$11937
  Bottom 0: 16.92,52.87 16.93,52.86
S$11938
  Bottom 0: 16.93,52.86 16.93,51.35
S$11939
  Bottom 0: 16.93,51.35 16.93,51.36
S$11940
  Bottom 0: 16.93,51.36 16.72,51.6
S$11941
  Bottom 0: 16.72,51.6 16.44,51.78
S$11942
  Bottom 0: 16.44,51.78 16.13,51.87
S$11943
  Bottom 0: 16.13,51.87 15.81,51.87
S$11944
  Bottom 0: 15.81,51.87 15.49,51.78
S$11945
  Bottom 0: 15.49,51.78 15.22,51.6
S$11946
  Bottom 0: 15.22,51.6 15.01,51.36
S$11947
  Bottom 0: 15.01,51.36 14.87,51.06
S$11948
  Bottom 0: 14.87,51.06 14.83,50.74
S$11949
  Bottom 0: 14.83,50.74 14.87,50.42
S$11950
  Bottom 0: 14.87,50.42 15.01,50.11
S$11951
  Bottom 0: 15.01,50.11 15.22,49.87
S$11952
  Bottom 0: 15.22,49.87 15.32,49.81
S$11953
  Bottom 0: 15.32,49.81 14.57,49.81
S$11954
  Bottom 0: 14.57,49.81 14.57,49.85
S$11955
  Bottom 0: 14.57,49.85 14.57,51.63
S$11956
  Bottom 0: 14.57,51.63 14.56,51.7
S$11957
  Bottom 0: 14.56,51.7 14.52,51.77
S$11958
  Bottom 0: 14.52,51.77 14.46,51.83
S$11959
  Bottom 0: 14.46,51.83 14.39,51.87
S$11960
  Bottom 0: 14.39,51.87 14.32,51.88
S$11961
  Bottom 0: 14.32,51.88 12.61,51.88
S$11962
  Bottom 0: 12.61,51.88 12.61,60.49
S$11963
  Bottom 0: 12.61,60.49 14.86,62.74
S$11964
  Bottom 0: 14.86,62.74 14.83,62.68
S$11965
  Bottom 0: 14.83,62.68 14.74,62.34
S$11966
  Bottom 0: 14.74,62.34 14.74,61.99
S$11967
  Bottom 0: 14.74,61.99 14.83,61.65
S$11968
  Bottom 0: 14.83,61.65 15,61.34
S$11969
  Bottom 0: 15,61.34 15.24,61.09
S$11970
  Bottom 0: 15.24,61.09 15.53,60.9
S$11971
  Bottom 0: 15.53,60.9 15.86,60.8
S$11972
  Bottom 0: 15.86,60.8 16.21,60.77
S$11973
  Bottom 0: 16.21,60.77 16.56,60.84
S$11974
  Bottom 0: 16.56,60.84 16.87,60.99
S$11975
  Bottom 0: 16.87,60.99 17.14,61.21
S$11976
  Bottom 0: 17.14,61.21 17.35,61.5
S$11977
  Bottom 0: 17.35,61.5 17.48,61.82
S$11978
  Bottom 0: 17.48,61.82 17.52,62.17
S$11979
  Bottom 0: 17.52,62.17 17.48,62.51
S$11980
  Bottom 0: 17.48,62.51 17.35,62.84
S$11981
  Bottom 0: 17.35,62.84 17.14,63.12
S$11982
  Bottom 0: 17.14,63.12 16.87,63.34
S$11983
  Bottom 0: 16.87,63.34 16.56,63.5
S$11984
  Bottom 0: 16.56,63.5 16.21,63.56
S$11985
  Bottom 0: 16.21,63.56 15.86,63.54
S$11986
  Bottom 0: 15.86,63.54 15.56,63.44
S$11987
  Bottom 0: 15.56,63.44 16.53,64.41
S$11988
  Bottom 0: 16.53,64.41 16.59,64.48
S$11989
  Bottom 0: 16.59,64.48 16.64,64.55
S$11990
  Bottom 0: 16.64,64.55 16.67,64.64
S$11991
  Bottom 0: 16.67,64.64 16.7,64.72
S$11992
  Bottom 0: 16.7,64.72 16.7,64.81
S$11993
  Bottom 0: 16.7,64.81 16.7,72
S$11994
  Bottom 0: 16.7,72 16.94,72.17
S$11995
  Bottom 0: 16.94,72.17 17.15,72.42
S$11996
  Bottom 0: 17.15,72.42 17.28,72.72
S$11997
  Bottom 0: 17.28,72.72 17.32,73.04
S$11998
  Bottom 0: 17.32,73.04 17.28,73.36
S$11999
  Bottom 0: 17.28,73.36 17.15,73.66
S$12000
  Bottom 0: 17.15,73.66 16.94,73.92
S$12001
  Bottom 0: 16.94,73.92 16.68,74.11
S$12002
  Bottom 0: 16.68,74.11 16.38,74.21
S$12003
  Bottom 0: 16.38,74.21 16.05,74.23
S$12004
  Bottom 0: 16.05,74.23 15.73,74.17
S$12005
  Bottom 0: 15.73,74.17 15.44,74.02
S$12006
  Bottom 0: 15.44,74.02 15.21,73.8
S$12007
  Bottom 0: 15.21,73.8 15.09,73.61
S$12008
  Bottom 0: 15.09,73.61 13.97,73.61
S$12009
  Bottom 0: 13.97,73.61 12.51,75.07
S$12010
  Bottom 0: 12.51,75.07 12.51,75.09
S$12011
  Bottom 0: 12.51,75.09 12.56,75.42
S$12012
  Bottom 0: 12.56,75.42 12.51,75.73
S$12013
  Bottom 0: 12.51,75.73 12.38,76.03
S$12014
  Bottom 0: 12.38,76.03 12.18,76.29
S$12015
  Bottom 0: 12.18,76.29 11.91,76.48
S$12016
  Bottom 0: 11.91,76.48 11.61,76.58
S$12017
  Bottom 0: 11.61,76.58 11.29,76.6
S$12018
  Bottom 0: 11.29,76.6 10.96,76.54
S$12019
  Bottom 0: 10.96,76.54 10.67,76.39
S$12020
  Bottom 0: 10.67,76.39 10.44,76.17
S$12021
  Bottom 0: 10.44,76.17 10.29,75.93
S$12022
  Bottom 0: 10.29,75.93 10.29,80.33
S$12023
  Bottom 0: 10.29,80.33 10.48,80.14
S$12024
  Bottom 0: 10.48,80.14 10.77,79.95
S$12025
  Bottom 0: 10.77,79.95 11.1,79.84
S$12026
  Bottom 0: 11.1,79.84 11.45,79.83
S$12027
  Bottom 0: 11.45,79.83 11.8,79.89
S$12028
  Bottom 0: 11.8,79.89 11.98,79.97
S$12029
  Bottom 0: 11.98,79.97 22.31,69.64
S$12030
  Bottom 0: 22.31,69.64 22.22,69.69
S$12031
  Bottom 0: 22.22,69.69 21.92,69.76
S$12032
  Bottom 0: 21.92,69.76 21.62,69.74
S$12033
  Bottom 0: 21.62,69.74 21.34,69.63
S$12034
  Bottom 0: 21.34,69.63 21.1,69.44
S$12035
  Bottom 0: 21.1,69.44 20.93,69.19
S$12036
  Bottom 0: 20.93,69.19 20.84,68.9
S$12037
  Bottom 0: 20.84,68.9 20.84,68.59
S$12038
  Bottom 0: 20.84,68.59 20.93,68.31
S$12039
  Bottom 0: 20.93,68.31 21.1,68.06
S$12040
  Bottom 0: 21.1,68.06 21.34,67.87
S$12041
  Bottom 0: 21.34,67.87 21.62,67.76
S$12042
  Bottom 0: 21.62,67.76 21.92,67.74
S$12043
  Bottom 0: 21.92,67.74 22.22,67.81
S$12044
  Bottom 0: 22.22,67.81 22.48,67.95
S$12045
  Bottom 0: 22.48,67.95 22.61,68.09
S$12046
  Bottom 0: 22.61,68.09 22.61,61.78
S$12047
  Bottom 0: 22.61,61.78 22.48,61.92
S$12048
  Bottom 0: 22.48,61.92 22.22,62.08
S$12049
  Bottom 0: 22.22,62.08 21.92,62.14
S$12050
  Bottom 0: 21.92,62.14 21.62,62.12
S$12051
  Bottom 0: 21.62,62.12 21.34,62.01
S$12052
  Bottom 0: 21.34,62.01 21.1,61.82
S$12053
  Bottom 0: 21.1,61.82 20.93,61.57
S$12054
  Bottom 0: 20.93,61.57 20.84,61.28
S$12055
  Bottom 0: 20.84,61.28 20.84,60.98
S$12056
  Bottom 0: 20.84,60.98 20.93,60.69
S$12057
  Bottom 0: 20.93,60.69 21.1,60.44
S$12058
  Bottom 0: 21.1,60.44 21.34,60.25
S$12059
  Bottom 0: 21.34,60.25 21.62,60.14
S$12060
  Bottom 0: 21.62,60.14 21.92,60.12
S$12061
  Bottom 0: 21.92,60.12 22.22,60.19
S$12062
  Bottom 0: 22.22,60.19 22.48,60.34
S$12063
  Bottom 0: 22.48,60.34 22.61,60.48
S$12064
  Bottom 0: 22.61,60.48 22.61,58.18
S$12065
  Bottom 0: 22.61,58.18 21.12,56.7
S$12066
  Bottom 0: 21.12,56.7 21.07,56.65
S$12067
  Bottom 0: 21.07,56.65 21.04,56.59
S$12068
  Bottom 0: 21.04,56.59 21.01,56.52
S$12069
  Bottom 0: 21.01,56.52 20.99,56.46
S$12070
  Bottom 0: 20.99,56.46 20.99,56.38
S$12071
  Bottom 0: 20.99,56.38 20.99,36.69
S$12072
  Bottom 0: 20.99,36.69 19.14,34.84
S$12073
  Bottom 0: 19.14,34.84 19.09,34.78
S$12074
  Bottom 0: 19.09,34.78 19.05,34.73
S$12075
  Bottom 0: 19.05,34.73 19.03,34.66
S$12076
  Bottom 0: 19.03,34.66 19.01,34.6
S$12077
  Bottom 0: 19.01,34.6 19,34.53
S$12078
  Bottom 0: 19,34.53 19,32.83
S$12079
  Bottom 0: 19,32.83 17.3,32.83
S$12080
  Bottom 0: 17.3,32.83 17.23,32.82
S$12081
  Bottom 0: 17.23,32.82 17.16,32.78
S$12082
  Bottom 0: 17.16,32.78 17.1,32.72
S$12083
  Bottom 0: 17.1,32.72 17.06,32.65
S$12084
  Bottom 0: 17.06,32.65 17.05,32.58
S$12085
  Bottom 0: 17.05,32.58 17.05,30.8
S$12086
  Bottom 0: 17.05,30.8 17.06,30.72
S$12087
  Bottom 0: 17.06,30.72 17.1,30.65
S$12088
  Bottom 0: 17.1,30.65 17.16,30.59
S$12089
  Bottom 0: 17.16,30.59 17.23,30.55
S$12090
  Bottom 0: 17.23,30.55 17.3,30.54
S$12091
  Bottom 0: 17.3,30.54 19.08,30.54
S$12092
  Bottom 0: 19.08,30.54 19.16,30.55
S$12093
  Bottom 0: 19.16,30.55 19.23,30.59
S$12094
  Bottom 0: 19.23,30.59
S$12095
  Bottom 0: 19.23,30.59 22.83,27
S$12096
  Bottom 0: 22.83,27 22.83,25.38
S$12097
  Bottom 0: 22.83,25.38 22.68,25.33
S$12098
  Bottom 0: 22.68,25.33 22.39,25.14
S$12099
  Bottom 0: 22.39,25.14 22.15,24.89
S$12100
  Bottom 0: 22.15,24.89 21.97,24.58
S$12101
  Bottom 0: 21.97,24.58 21.89,24.24
S$12102
  Bottom 0: 21.89,24.24 21.89,23.89
S$12103
  Bottom 0: 21.89,23.89 21.97,23.55
S$12104
  Bottom 0: 21.97,23.55 22.15,23.24
S$12105
  Bottom 0: 22.15,23.24 22.39,22.99
S$12106
  Bottom 0: 22.39,22.99 22.68,22.8
S$12107
  Bottom 0: 22.68,22.8 23.01,22.7
S$12108
  Bottom 0: 23.01,22.7 23.36,22.68
S$12109
  Bottom 0: 23.36,22.68 23.43,22.68
S$12110
  Bottom 0: 23.43,22.68 13.95,13.21
S$12111
  Bottom 0: 13.95,13.21 12.19,13.21
S$12112
  Bottom 0: 17.01,20.14 17.35,20.2
S$12113
  Bottom 0: 17.35,20.2 17.67,20.35
S$12114
  Bottom 0: 17.67,20.35 17.94,20.57
S$12115
  Bottom 0: 17.94,20.57 18.15,20.86
S$12116
  Bottom 0: 18.15,20.86 18.27,21.18
S$12117
  Bottom 0: 18.27,21.18 18.32,21.53
S$12118
  Bottom 0: 18.32,21.53 18.27,21.87
S$12119
  Bottom 0: 18.27,21.87 18.15,22.2
S$12120
  Bottom 0: 18.15,22.2 17.94,22.48
S$12121
  Bottom 0: 17.94,22.48 17.67,22.7
S$12122
  Bottom 0: 17.67,22.7 17.35,22.86
S$12123
  Bottom 0: 17.35,22.86 17.01,22.92
S$12124
  Bottom 0: 17.01,22.92 16.66,22.9
S$12125
  Bottom 0: 16.66,22.9 16.33,22.79
S$12126
  Bottom 0: 16.33,22.79 16.04,22.6
S$12127
  Bottom 0: 16.04,22.6 15.8,22.35
S$12128
  Bottom 0: 15.8,22.35 15.62,22.04
S$12129
  Bottom 0: 15.62,22.04 15.54,21.7
S$12130
  Bottom 0: 15.54,21.7 15.54,21.35
S$12131
  Bottom 0: 15.54,21.35 15.62,21.01
S$12132
  Bottom 0: 15.62,21.01 15.8,20.7
S$12133
  Bottom 0: 15.8,20.7 16.04,20.45
S$12134
  Bottom 0: 16.04,20.45 16.33,20.26
S$12135
  Bottom 0: 16.33,20.26 16.66,20.16
S$12136
  Bottom 0: 16.66,20.16 17.01,20.14
S$12137
  Bottom 0: 19.46,24.32 19.91,24.37
S$12138
  Bottom 0: 19.91,24.37 20.34,24.49
S$12139
  Bottom 0: 20.34,24.49 20.73,24.71
S$12140
  Bottom 0: 20.73,24.71 21.08,24.99
S$12141
  Bottom 0: 21.08,24.99 21.36,25.34
S$12142
  Bottom 0: 21.36,25.34 21.57,25.73
S$12143
  Bottom 0: 21.57,25.73 21.7,26.16
S$12144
